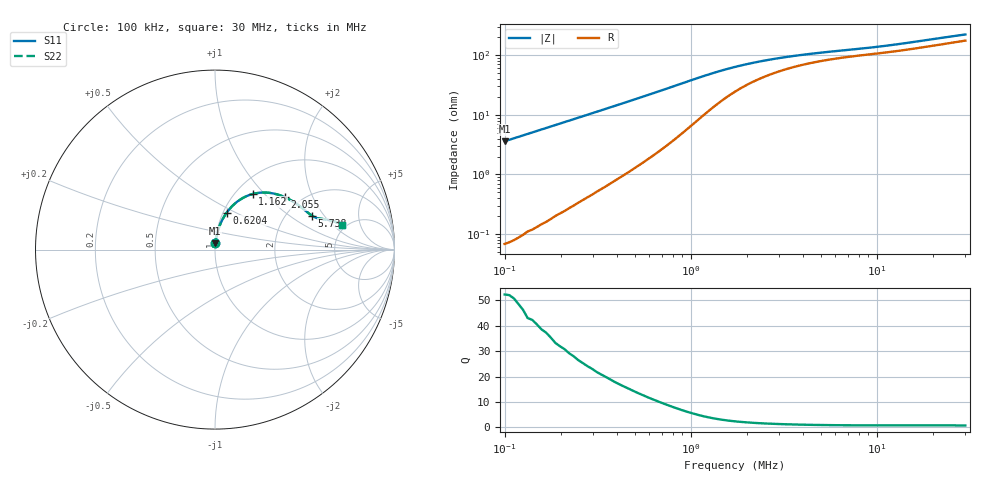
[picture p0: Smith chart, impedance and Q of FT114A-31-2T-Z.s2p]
! ListType=Log
!!FT114A-31 2T Z
# MHZ S RI R 50
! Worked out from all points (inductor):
!   101 points, 100 kHz to 30 MHz, reference 50 ohm
!   read as one part in series: L = 5.72 uH near 100 kHz
!   highest Q = 52.3 at 100 kHz (marker M1), where L = 5.72 uH
!   S11 on the Smith chart (normalised r, x): 100 kHz: 1.00, +0.07; 620.4 kHz: 1.04, +0.45; 1.162 MHz: 1.19, +0.86; 2.055 MHz: 1.66, +1.27; 5.738 MHz: 2.71, +1.53; 30 MHz: 4.59, +2.63
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0.1  0.00209 0.0358  0.9981 -0.0359  0.9981 -0.0359  0.00207 0.0358
0.1670863  0.00533 0.0596  0.995 -0.0597  0.995 -0.0596  0.00532 0.0595
0.2637003  0.0126 0.0931  0.9876 -0.0932  0.9876 -0.0931  0.0126 0.0929
0.350725  0.0218 0.1225  0.9784 -0.1226  0.9785 -0.1225  0.0218 0.1223
0.4406071  0.0338 0.1518  0.9664 -0.152  0.9665 -0.1518  0.0338 0.1516
0.62041  0.0656 0.2064  0.9347 -0.2067  0.9348 -0.2065  0.0654 0.2061
0.6953784  0.0818 0.227  0.9184 -0.2274  0.9187 -0.2272  0.0816 0.2267
0.8735868  0.1265 0.2691  0.8736 -0.2696  0.874 -0.2693  0.1263 0.2688
0.9791484  0.1562 0.2881  0.844 -0.2887  0.8444 -0.2884  0.1558 0.2879
1.161882  0.2092 0.3096  0.7911 -0.3102  0.7915 -0.31  0.2087 0.3094
1.459644  0.2869 0.3176  0.7132 -0.3183  0.7138 -0.3183  0.2863 0.3176
1.833715  0.358 0.3039  0.6422 -0.3048  0.6427 -0.305  0.3575 0.3041
2.055296  0.3882 0.2923  0.612 -0.2932  0.6124 -0.2934  0.3878 0.2925
2.438866  0.4267 0.2725  0.5734 -0.2734  0.5737 -0.2737  0.4264 0.2727
2.89402  0.4582 0.252  0.5419 -0.2532  0.5421 -0.2535  0.458 0.2523
3.635686  0.4915 0.2269  0.5085 -0.2283  0.5087 -0.2285  0.4914 0.2271
4.567423  0.5176 0.2058  0.4824 -0.2075  0.4825 -0.2077  0.5175 0.206
5.737941  0.5392 0.1899  0.4607 -0.1919  0.4608 -0.1921  0.5391 0.19
8.079479  0.5685 0.1756  0.4313 -0.1784  0.4314 -0.1785  0.5685 0.1757
12.04431  0.6075 0.1692  0.392 -0.1732  0.3922 -0.1732  0.6075 0.1693
17.95479  0.6533 0.1598  0.3459 -0.1654  0.346 -0.1655  0.6532 0.1599
30  0.7071 0.1381  0.2914 -0.1468  0.2914 -0.1469  0.7071 0.1382
